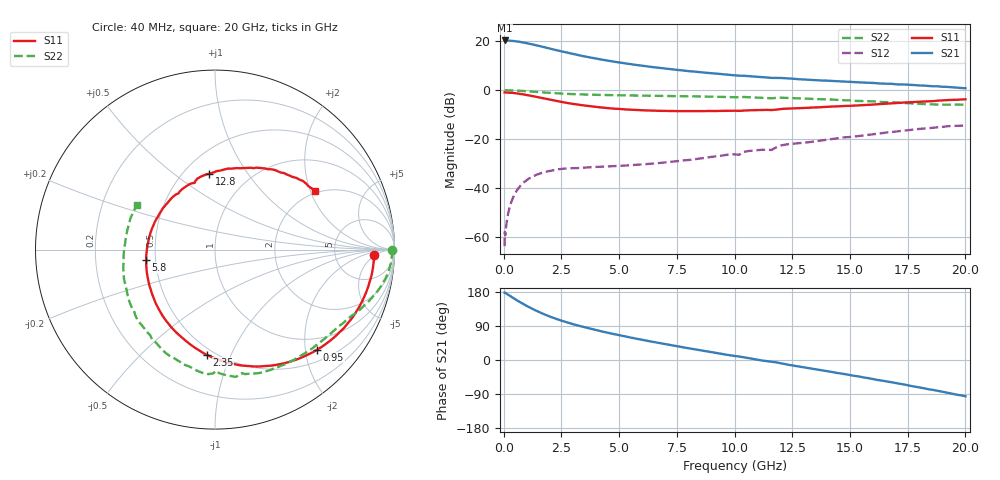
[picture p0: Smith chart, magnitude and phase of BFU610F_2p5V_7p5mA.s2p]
! Filename:  P:\Prog\Test\Noise\ATS_data\Testdata_Net\SplitFiles\BFU610_2W_A5_HighFreq_2.5V_7.5mA_D.s2p
! Date/Time: Wed 10/Aug/2011 16:55:31
! BFU610_2W_A5_HighFreq_Bias5_2.5V_1mA_10mA_R.s2p
! MDIF S-parameter v. bias file
! BFU610_2W_A5_HighFreq_2.5V_1mA_10mA
! Date/time Mon Aug 08 14:04:20 2011
! VAR V_out= 2.5000
! VAR I_out= 7.5000
! VAR V_in= 0.9119
! VAR I_in= 0.0648
! Device data file deembeded for feedlines and parallel
! Original file: \SplitFiles\BFU610_2W_A5_HighFreq_2.5V_7.5mA_R.s2p
! Feed-files: PR003V01_101208_Feed1.s2p, PR003V01_101208_Feed2.s2p
! Parallel-file: PR003V01_101208_Par.s2p
# MHz S MA R 50
!  Freq-MHz  S11-mag  S11-arg  S21-mag  S21-arg  S12-mag  S12-arg  S22-mag  S22-arg
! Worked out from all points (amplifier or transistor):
!   167 points, 40 MHz to 20 GHz, reference 50 ohm
!   highest |S21| = 20.3 dB at 40 MHz (marker M1)
!   |S21| within 3 dB of that: start of sweep to 1.867 GHz
!   unconditionally stable (mu >= 1): 3.305 GHz to end of sweep
!   at 550 MHz: K = 0.14, MSG = 30.7 dB, |S12| = -41.5 dB
!   at 4.2 GHz: K = 1.27, MAG = 18.9 dB, |S12| = -31.4 dB
!   at 20 GHz: K = 1.05, MAG = 6.3 dB, |S12| = -14.5 dB
!   S11 on the Smith chart (normalised r, x): 40 MHz: 16, -4; 950 MHz: 0.74, -2.25; 2.35 GHz: 0.46, -0.82; 5.8 GHz: 0.44, -0.06; 12.8 GHz: 0.66, +0.68; 20 GHz: 1.93, +2.15
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40  0.8875 -1.9  10.32 178.1  0.0006342 87.0  0.9842 -0.2
50  0.8845 -2.2  10.28 178.0  0.001247 98.7  0.9849 -0.4
70  0.8875 -3.3  10.26 177.1  0.001063 87.6  0.9863 -0.7
260  0.8797 -12.7  10.22 169.7  0.004018 85.5  0.9844 -3.6
400  0.8687 -19.5  10.09 164.2  0.006191 81.0  0.9796 -5.6
700  0.8336 -33.4  9.648 152.9  0.01058 72.5  0.9631 -9.7
950  0.797 -44.4  9.188 144.3  0.01373 66.2  0.9458 -12.7
1250  0.7497 -56.6  8.561 134.8  0.01688 59.4  0.923 -15.9
1500  0.709 -66.2  8.046 127.5  0.01898 54.6  0.9055 -18.3
1950  0.6407 -81.9  7.149 115.8  0.02182 47.8  0.8764 -22.1
2350  0.5882 -94.5  6.413 107.0  0.02375 43.9  0.8496 -25.3
2900  0.5272 -109.5  5.588 96.4  0.02497 38.0  0.8279 -28.9
3400  0.4878 -122.1  4.976 88.1  0.02555 36.9  0.8107 -32.2
4400  0.4297 -144.4  4.068 73.3  0.027 35.8  0.7889 -38.6
5800  0.3877 -171.5  3.227 55.6  0.02943 38.5  0.767 -47.9
6800  0.3737 171.3  2.81 44.1  0.03219 41.4  0.7545 -54.7
8800  0.3706 141.2  2.244 22.6  0.04114 46.0  0.7328 -69.0
10200  0.3734 122.7  1.958 9.2  0.04709 48.7  0.707 -78.1
12800  0.4244 94.6  1.655 -17.2  0.08171 39.9  0.6699 -101.5
13400  0.438 88.5  1.595 -23.2  0.08753 37.0  0.6548 -107.4
16800  0.5316 58.2  1.337 -59.0  0.1377 15.1  0.5573 -149.1
20000  0.6447 30.3  1.083 -95.7  0.188 -17.2  0.5011 150.5
